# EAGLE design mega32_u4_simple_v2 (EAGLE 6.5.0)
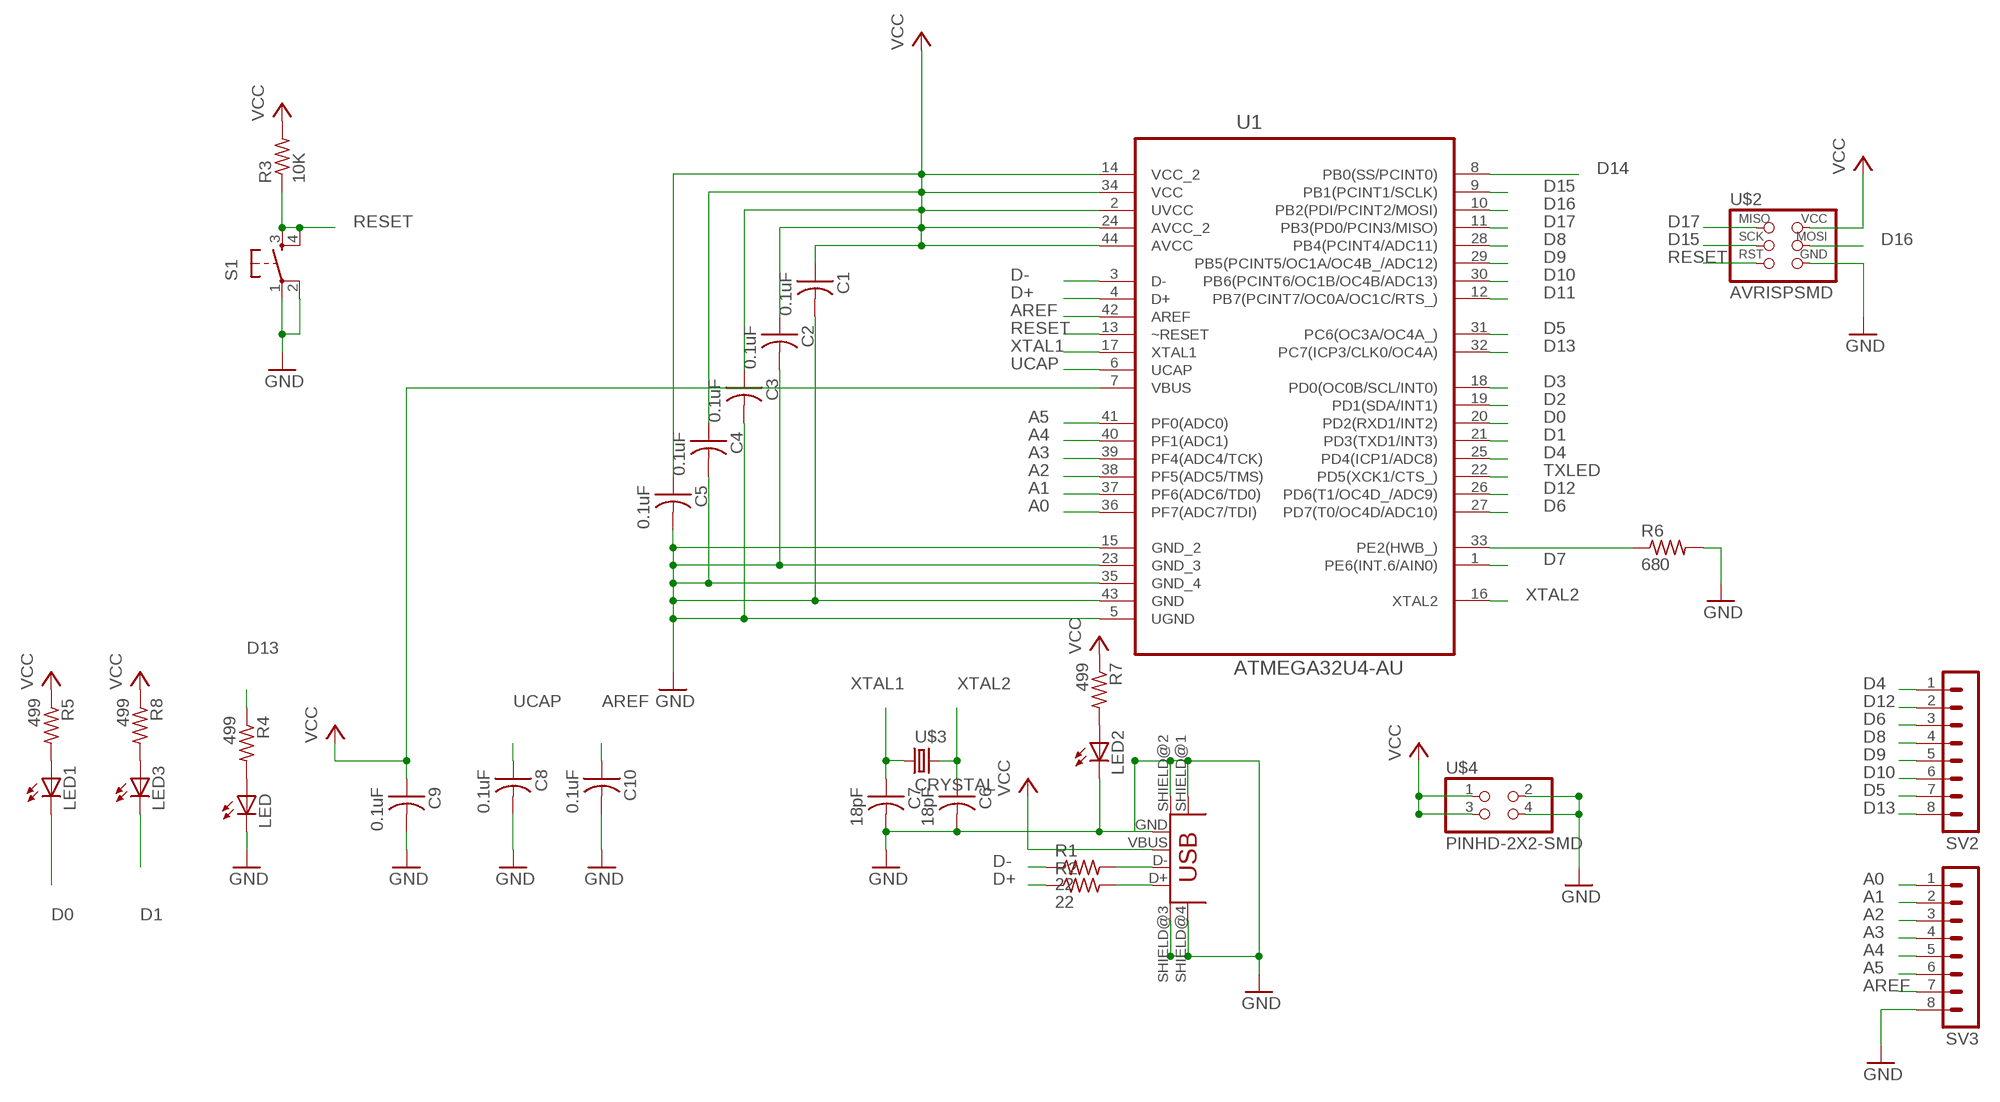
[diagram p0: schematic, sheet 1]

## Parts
C1  0.1uF  CAP-US1206FAB  [C1206FAB]
C2  0.1uF  CAP-US1206FAB  [C1206FAB]
C3  0.1uF  CAP-US1206FAB  [C1206FAB]
C4  0.1uF  CAP-US1206FAB  [C1206FAB]
C5  0.1uF  CAP-US1206FAB  [C1206FAB]
C6  18pF  CAP-US1206FAB  [C1206FAB]
C7  18pF  CAP-US1206FAB  [C1206FAB]
C8  0.1uF  CAP-US1206FAB  [C1206FAB]
C9  0.1uF  CAP-US1206FAB  [C1206FAB]
C10  0.1uF  CAP-US1206FAB  [C1206FAB]
LED  LED1206  [1206]
LED1  LED1206  [1206]
LED2  LED1206  [1206]
LED3  LED1206  [1206]
R1  22  RES-US1206FAB  [R1206FAB]
R2  22  RES-US1206FAB  [R1206FAB]
R3  10K  RES-US1206FAB  [R1206FAB]
R4  499  RESISTOR1206  [1206]
R5  499  RESISTOR1206  [1206]
R6  680  RES-US1206FAB  [R1206FAB]
R7  499  RESISTOR1206  [1206]
R8  499  RESISTOR1206  [1206]
S1  6MM_SWITCH6MM_SWITCH  [6MM_SWITCH]
SV2  MA08-1  [MA08-1]
SV3  MA08-1  [MA08-1]
U1  ATMEGA32U4-AU  [QFP80P1200X1200X120-44N]
U$1  USB_MINIB  [USB_MINIB]
U$2  AVRISPSMD  [2X03SMD]
U$3  CRYSTAL  [2-SMD-5X3MM]
U$4  PINHD-2X2-SMD  [2X02SMD]

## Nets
A0: SV3.1 U1.36(PF7(ADC7/TDI))
A1: SV3.2 U1.37(PF6(ADC6/TD0))
A2: SV3.3 U1.38(PF5(ADC5/TMS))
A3: SV3.4 U1.39(PF4(ADC4/TCK))
A4: SV3.5 U1.40(PF1(ADC1))
A5: SV3.6 U1.41(PF0(ADC0))
AREF: C10.1 SV3.7 U1.42(AREF)
D0: LED1.2(C) U1.20(PD2(RXD1/INT2))
D1: LED3.2(C) U1.21(PD3(TXD1/INT3))
D2: U1.19(PD1(SDA/INT1))
D3: U1.18(PD0(OC0B/SCL/INT0))
D4: SV2.1 U1.25(PD4(ICP1/ADC8))
D5: SV2.7 U1.31(PC6(OC3A/OC4A_))
D6: SV2.3 U1.27(PD7(T0/OC4D/ADC10))
D7: U1.1(PE6(INT.6/AIN0))
D8: SV2.4 U1.28(PB4(PCINT4/ADC11))
D9: SV2.5 U1.29(PB5(PCINT5/OC1A/OC4B_/ADC12))
D10: SV2.6 U1.30(PB6(PCINT6/OC1B/OC4B/ADC13))
D11: U1.12(PB7(PCINT7/OC0A/OC1C/RTS_))
D12: SV2.2 U1.26(PD6(T1/OC4D_/ADC9))
D13: R4.1 SV2.8 U1.32(PC7(ICP3/CLK0/OC4A))
D14: U1.8(PB0(SS/PCINT0))
D15: U1.9(PB1(PCINT1/SCLK)) U$2.3(SCK)
D16: U1.10(PB2(PDI/PCINT2/MOSI)) U$2.4(MOSI)
D17: U1.11(PB3(PD0/PCIN3/MISO)) U$2.1(MISO)
D+: R2.1 U1.4(D+)
D-: R1.1 U1.3(D-)
GND: C1.2 C2.2 C3.2 C4.2 C5.2 C6.2 C7.2 C8.2 C9.2 C10.2 LED2.2(C) LED.2(C) R6.2 S1.1(P) S1.2(P1) SV3.8 U1.5(UGND) U1.15(GND_2) U1.23(GND_3) U1.35(GND_4) U1.43(GND) U$1.GND U$1.SHIELD@1(SHIELD) U$1.SHIELD@2(SHIELD1) U$1.SHIELD@3(SHIELD2) U$1.SHIELD@4(SHIELD3) U$2.6(GND) U$4.2 U$4.4
N$1: R1.2 U$1.D-
N$2: R2.2 U$1.D+
N$3: LED.1(A) R4.2
N$4: LED1.1(A) R5.2
N$5: LED2.1(A) R7.2
N$6: LED3.1(A) R8.2
N$35: R6.1 U1.33(PE2(HWB_))
RESET: R3.1 S1.3(S) S1.4(S1) U1.13(~RESET) U$2.5(RST)
TXLED: U1.22(PD5(XCK1/CTS_))
UCAP: C8.1 U1.6(UCAP)
VCC: C1.1 C2.1 C3.1 C4.1 C5.1 C9.1 R3.2 R5.1 R7.1 R8.1 U1.2(UVCC) U1.7(VBUS) U1.14(VCC_2) U1.24(AVCC_2) U1.34(VCC) U1.44(AVCC) U$1.VBUS U$2.2(VCC) U$4.1 U$4.3
XTAL1: C7.1 U1.17(XTAL1) U$3.P$1
XTAL2: C6.1 U1.16(XTAL2) U$3.P$2

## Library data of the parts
C1-C10 = fab:CAP-US
LED LED1-LED3 = ng:LED
R1-R3 R6 = fab:RES-US: Resistor (US Symbol)
R4 R5 R7 R8 = ng:RESISTOR
S1 = ng:6MM_SWITCH: OMRON SWITCH
SV2 SV3 = con-lstb:MA08-1: PIN HEADER
U1 = Atmel_By_element14_Batch_1:ATMEGA32U4-AU: 8-bit Microcontroller with ISP Flash and USB Controller; MPN: ATMEGA32U4-AU; OC_FARNELL: 1748525; OC_NEWARK: 26R5633; PACKAGE: TQFP-44; SUPPLIER: Atmel
U$1 = fab:USB_MINIB
U$2 = fab:AVRISP
U$3 = fab:CRYSTAL
U$4 = fab:PINHD-2X2-SMD

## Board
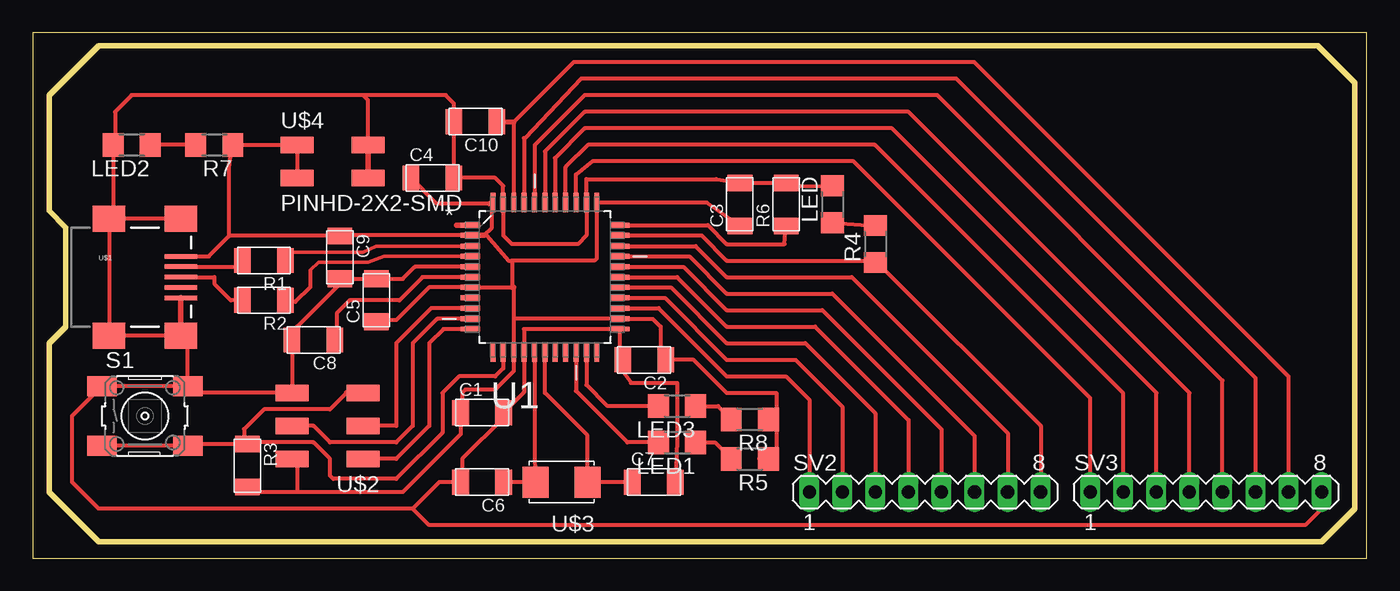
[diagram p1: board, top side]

Size 102.54 x 40.38 mm. Coordinates in mm from the lower left corner, seen from the top.
Outline: 0,0 102.54,0 102.54,40.38 0,40.38 0,0
Copper layers (1*16): Top 0.035mm / dielectric 1.5mm / Bottom 0.035mm
Design rules "default *": minimum track width 10mil, minimum drill 24mil, track to track 0.4mm, track to pad 0.4mm, pad to pad 0.4mm, via to via 0.4mm, smd to smd 0.4mm, copper to edge 40mil, drill to drill 0.4mm, minimum pad ring 10mil, minimum via ring 8mil, stop-mask expansion 4mil, vias tented up to drill 0mil, thermal gap 10mil
Milling: area 1.3,1.3 to 101.6,39.4

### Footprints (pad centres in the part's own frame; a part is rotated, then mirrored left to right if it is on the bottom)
C1206FAB = smd 1.27 x 1.905: 1 -1.651,0; 2 1.651,0
1206 = smd 1.6 x 1.803: 1 -1.422,0; 2 1.422,0
R1206FAB = smd 1.27 x 1.905: 1 -1.651,0; 2 1.651,0
6MM_SWITCH = smd 2.286 x 1.524: 1 -3.302,2.286; 2 3.302,2.286; 3 -3.302,-2.286; 4 3.302,-2.286
MA08-1 = drill 1.016 long: 1 -8.89,0; 2 -6.35,0; 3 -3.81,0; 4 -1.27,0; 5 1.27,0; 6 3.81,0; 7 6.35,0; 8 8.89,0
QFP80P1200X1200X120-44N = smd 1.5 x 0.38: 1 -5.74,3.988; 2 -5.74,3.2; 3 -5.74,2.388; 4 -5.74,1.6; 5 -5.74,0.787; 6 -5.74,0; 7 -5.74,-0.787; 8 -5.74,-1.6; 9 -5.74,-2.388; 10 -5.74,-3.2; 11 -5.74,-3.988; 23 5.74,-3.988; 24 5.74,-3.2; 25 5.74,-2.388; 26 5.74,-1.6; 27 5.74,-0.787; 28 5.74,0; 29 5.74,0.787; 30 5.74,1.6; 31 5.74,2.388; 32 5.74,3.2; 33 5.74,3.988 | smd 0.38 x 1.5: 12 -3.988,-5.74; 13 -3.2,-5.74; 14 -2.388,-5.74; 15 -1.6,-5.74; 16 -0.787,-5.74; 17 0,-5.74; 18 0.787,-5.74; 19 1.6,-5.74; 20 2.388,-5.74; 21 3.2,-5.74; 22 3.988,-5.74; 34 3.988,5.74; 35 3.2,5.74; 36 2.388,5.74; 37 1.6,5.74; 38 0.787,5.74; 39 0,5.74; 40 -0.787,5.74; 41 -1.6,5.74; 42 -2.388,5.74; 43 -3.2,5.74; 44 -3.988,5.74
USB_MINIB = smd 2.5 x 0.35: D+ 3.77,0; D- 3.77,0.8; GND 3.77,-1.6; ID 3.77,-0.8; VBUS 3.77,1.6 | smd 2.5 x 2: SHIELD@1 -1.73,-4.5; SHIELD@2 -1.73,4.5; SHIELD@3 3.77,4.5; SHIELD@4 3.77,-4.5
2X03SMD = smd 2.54 x 1.27: 1 -2.54,2.54; 2 2.92,2.54; 3 -2.54,0; 4 2.92,0; 5 -2.54,-2.54; 6 2.92,-2.54
2-SMD-5X3MM = smd 2 x 2.4: P$1 -2,0; P$2 2,0
2X02SMD = smd 2.54 x 1.27: 1 -2.54,1.27; 2 2.92,1.27; 3 -2.54,-1.27; 4 2.92,-1.27

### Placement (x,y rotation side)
C1  34.54,11.18 0 top
C2  46.99,15.24 180 top
C3  54.36,27.18 90 top
C4  30.73,29.21 0 top
C5  26.42,19.81 90 top
C6  34.54,5.84 180 top
C7  47.75,5.84 0 top
C8  21.59,16.76 180 top
C9  23.62,23.11 270 top
C10  34.04,33.53 180 top
LED  61.47,27.18 90 top
LED1  49.53,8.89 180 top
LED2  7.62,31.75 180 top
LED3  49.53,11.68 180 top
R1  17.78,22.86 180 top
R2  17.78,19.81 180 top
R3  16.51,7.11 270 top
R4  64.77,24.13 90 top
R5  55.12,7.62 180 top
R6  57.91,27.18 90 top
R7  13.97,31.75 180 top
R8  55.12,10.67 180 top
S1  8.64,10.92 0 top
SV2  68.58,5.08 0 top
SV3  90.17,5.08 0 top
U1  39.37,21.59 0 top
U$1  7.62,21.59 0 top
U$2  22.86,10.16 180 top
U$3  40.64,5.84 180 top
U$4  22.86,30.48 0 top

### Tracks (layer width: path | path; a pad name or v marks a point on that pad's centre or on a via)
A0
  Top 0.305: U1.36 41.76,29.46 43.03,30.48 63.1,30.48 81.28,12.3 SV3.1
A1
  Top 0.305: U1.37 40.97,30.05 42.67,31.75 64.73,31.75 83.82,12.66 SV3.2
A2
  Top 0.305: SV3.3 86.36,12.7 66.04,33.02 42.42,33.02 40.13,30.73 40.16,30.73 U1.38
A3
  Top 0.305: SV3.4 88.9,12.7 67.31,34.29 42.42,34.29 39.37,31.24 U1.39
A4
  Top 0.305: SV3.5 91.44,13.64 69.52,35.56 42.42,35.56 38.61,31.75 38.58,31.75 U1.40
A5
  Top 0.305: SV3.6 93.98,13.83 70.98,36.83 42.16,36.83 37.85,32.26 37.77,32.26 U1.41
AREF
  Top 0.305: SV3.7 96.52,13.94 72.36,38.1 41.58,38.1 36.98,33.5 U1.42
  Top 0.406: 36.98,33.5 C10.1
D0
  Top 0.305: U1.20 41.76,12.85 45.72,8.89 LED1.2
D1
  Top 0.305: U1.21 42.57,13.31 44.2,11.68 LED3.2
D4
  Top 0.305: U1.25 48.11,19.2 53.34,13.97 57.89,13.97 59.69,12.17 SV2.1
D5
  Top 0.305: U1.31 50.95,23.98 53.34,21.59 62.95,21.59 74.93,9.61 | 74.93,9.61 SV2.7 74.93,9.61
D6
  Top 0.305: U1.27 49.05,20.8 53.34,16.51 59.38,16.51 64.77,11.12 SV2.3
D7
  Top 0.406: U1.1 32.59,25.58
D8
  Top 0.305: U1.28 49.53,21.59 53.34,17.78 60.13,17.78 67.31,10.6 SV2.4
D9
  Top 0.305: U1.29 50.01,22.38 53.34,19.05 60.69,19.05 69.85,9.89 SV2.5
D10
  Top 0.305: U1.30 50.47,23.19 53.34,20.32 61.46,20.32 72.39,9.39 SV2.6
D12
  Top 0.305: U1.26 48.59,19.99 53.34,15.24 58.64,15.24 62.23,11.65 SV2.2
D13
  Top 0.305: U1.32 51.41,24.79 53.34,22.86 64.62,22.86 | 64.92,22.71 77.47,10.16 | 77.47,10.16 SV2.8 | 77.47,10.16 SV2.8 | 77.47,10.16 SV2.8
  Top 0.406: 64.62,22.86 R4.1 64.92,22.71
D15
  Top 0.305: U1.9 30.63,19.2 27.94,16.51 27.94,10.16 U$2.3
D16
  Top 0.305: U1.10 31.09,18.39 29.21,16.51 29.21,10.16 27.94,8.89 22.86,8.89 21.59,10.16 U$2.4
D17
  Top 0.305: U1.11 31.57,17.6 30.48,16.51 30.48,10.16 27.94,7.62 U$2.1
D+
  Top 0.254: U1.4 27,23.19 25.78,22.73 21.97,22.73 21.34,22.1
  Top 0.305: 21.34,22.1 21.34,20.83 20.19,19.69 19.56,19.69 R2.1
D-
  Top 0.254: U1.3 26.39,23.98 25.4,23.5 19.56,23.5
  Top 0.305: 19.56,23.5 19.3,22.99 R1.1
GND
  Top 0.305: U$1.SHIELD@4 U$1.SHIELD@1 U$1.SHIELD@2 U$1.SHIELD@3 | U1.5 29.36,22.38 28.45,21.46 C5.2 C9.2 | LED2.2 6.2,26.4 | R6.2 C3.2 52.55,29.11 42.57,29.11 U1.35 42.57,24.79 41.91,24.13 36.83,24.13 36.17,24.79 U1.43 36.17,28.6 35.56,29.21 C4.2 C10.2 32.38,34.93 31.75,35.56 25.4,35.56 | 58.9,28.57 LED.2 | 45.11,15.47 U1.23 37.77,17.6 U1.15 37.77,12.75 C1.2 | C2.2 45.34,14.35 45.97,13.46 49.53,13.46 49.53,9.02 C7.2 | U$2.6 11.94,12.7 | C8.2 U$2.6 | 11.94,16.54 S1.2 S1.1 3.05,10.92 3.05,5.84 5.08,3.81 29.21,3.81 | 36.2,10.8 33.02,7.62 33.02,5.97 | C6.2 31.24,5.84 29.21,3.81 | 25.4,35.56 7.62,35.56 6.35,34.29 6.35,31.9 | U$4.4 25.78,35.18 25.4,35.56 | SV3.8 99.06,3.81 97.79,2.54 30.48,2.54 29.21,3.81 | 23.62,21.08 20.32,17.78 20.32,17.14
  Top 0.406: U$1.GND U$1.SHIELD@4 11.94,16.54 | U$1.SHIELD@3 11.43,26.09 | 6.2,26.4 U$1.SHIELD@2 | R6.2 58.9,28.57 | 45.11,15.47 C2.2 | 11.94,12.7 S1.2 | U$4.2 U$4.4 | C9.2 23.62,21.08 | 20.32,17.14 C8.2 | U$2.6 | C1.2 36.2,10.8 | 33.02,5.97 C6.2 | 6.35,31.9 LED2.2
N$1
  Top 0.305: U$1.D- 16.13,22.39
  Top 0.406: 16.13,22.39 R1.2
N$2
  Top 0.305: R2.2 15.24,19.81 13.97,21.08 13.97,21.59 U$1.D+
N$3
  Top 0.305: LED.1 R4.2
N$4
  Top 0.305: LED1.1 52.43,8.89 R5.2
N$5
  Top 0.305: R7.2 LED2.1
N$6
  Top 0.305: LED3.1 52.68,11.68 R8.2
N$35
  Top 0.305: U1.33 51.89,25.58 53.34,24.13 57.79,24.13 R6.1
RESET
  Top 0.305: S1.4 S1.3 | U1.13 36.17,14.58 35.56,13.97 32.77,13.97 31.5,12.7 31.5,9.65 27.94,6.1 23.11,6.1 22.86,6.35 22.86,7.62 21.59,8.89 16.64,8.89 | 24.13,12.7 22.86,11.43 17.78,11.43 16.26,9.91 16.26,9.02 R3.1 11.94,8.76
  Top 0.406: 16.64,8.89 R3.1 | U$2.5 24.13,12.7 | 11.94,8.76 S1.4
UCAP
  Top 0.305: U1.6 29.97,21.59 28.19,19.81 24.38,19.81 23.37,18.8 23.37,16.89 C8.1
VCC
  Top 0.305: 34.7,24.79 35.31,25.4 35.31,27.25 | 23.65,24.79 U1.2 34.9,24.79 36.58,22.86 36.83,22.86 | C9.1 15.11,24.77 | 15.11,24.77 13.54,23.19 U$1.VBUS | 15.11,24.77 15.11,30.2 R7.1 U$4.1 U$4.3 | C3.1 51.79,27.33 U1.34 43.36,23.04 43.18,22.86 36.83,22.86 | 48.26,15.62 48.26,17.78 47.65,18.39 U1.24 36.98,18.39 | 35.13,27.23 31.06,27.23 C4.1 | C2.1 50.8,15.24 53.34,12.7 57.15,12.7 57.15,10.31 57.15,7.62 | 33.02,11.3 33.02,12.7 33.27,12.95 35.56,12.95 36.98,14.38 U1.14 36.98,18.39 | 20.32,5.08 16.89,5.08 R3.2 | 20.32,7.62 20.32,5.08 | C1.1 32.89,9.52 28.45,5.08 20.32,5.08 | 36.98,20.8 36.98,18.39 | 36.83,22.86 36.83,20.8 U1.7 30.45,20.8 27.94,18.29 26.04,18.29 C5.1
  Top 0.406: U1.2 34.7,24.79 | 35.31,27.25 U1.44 35.13,27.23 | 43.43,27.25 U1.34 | 23.65,24.79 C9.1 | 29.21,29.08 C4.1 | 48.26,15.62 C2.1 | 57.15,10.31 R8.1 | 57.15,7.62 R5.1 55.88,7.62 | 33.02,11.3 C1.1 | U$2.2 20.32,7.62 | 36.83,20.8 36.98,20.8
XTAL1
  Top 0.305: C7.1 U$3.P$1 42.64,9.43 39.37,12.7 U1.17
XTAL2
  Top 0.305: C6.1 U$3.P$2 38.58,7.68 U1.16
